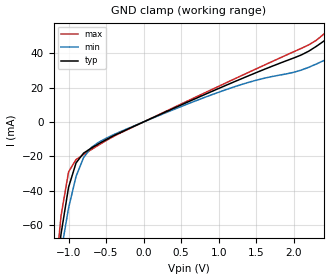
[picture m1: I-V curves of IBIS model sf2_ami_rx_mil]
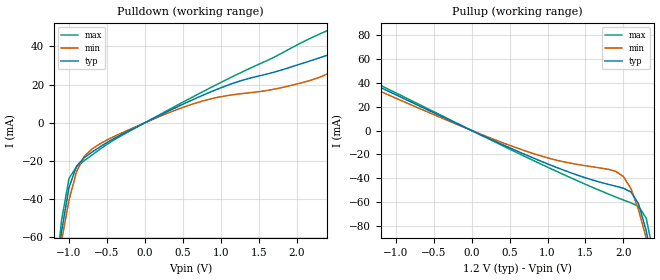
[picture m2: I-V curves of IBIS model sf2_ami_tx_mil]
|   Microsemi Corporation
|   SmarFusion2/IGLOO2 Military IBIS-AMI Models
[IBIS ver]   5.0
[File name]   sf2_igl2_ami_mil.ibs
[File Rev]   1.3
[Date]   February 1, 2019
[Disclaimer] These IBIS Models are Provided "As is" with NO WARRANTY
   whatsoever and signal integrity software specifically disclaims any
   implied warranties of merchantability, fitness for a particular
   purpose or against infringement.
[Source]   Original model developed in collaboration with Sigrity. Optimized by SiSoft.
[Notes]   Known limitations: Main tap is limited to maximum amplitude setting only
   and cannot be adjusted.
-Revision History:
1.4: February 1, 2019
   * Added model limitation note on abicdr_tx.ami and sf2_igl2_ami_mil.ibs files.
1.3: July 22, 2015
   * Added Algorithmic Model to support 64-bit Window environment
1.2: April 2, 2015
   * Added new RLC packages in Package section.
1.1: June 12, 2014
   * Updated Package section.
   * Consolidated the IGLOO2 and SmartFusion2 IBIS AMI Model
   * Updated the RX .ami model to clarify comments.
1.05: 6 November 2013
   Based on the model 1.0 model supplied by Microsemi dated 18 March 2013.
   This model has been optimized for use with SiSoft's QCD Simulator. Points of note:
   * Updated [Ramp] data to correct single-ended / differential issues
   * Updated C_comp values using data provided by Microsemi
   * Updated TX .ami file to disable auto EQ mode (does not work with QCD)
   * Included TX jitter data derived from PCIe Gen2 compliance testing
   * Signed models as QCD Certified
1.0: 18 March 2013 20:52:13
   * Original model supplied by Microsemi
[Copyright]  (c) 2013, Microsemi Corporation, All Rights Reserved.
[Component]  SF2_IGL2_ibis_ami_mil
[Manufacturer] Microsemi Corporation
[Package]
|   typ   min   max
| M2S/M2GL010
|R_pkg   0.66635   0.053835   1.0211   |010-FG484
|L_pkg   5.248e-9   6.178e-10   7.432e-9   |010-FG484
|C_pkg   1.306e-12   8.624e-13   3.748e-12   |010-FG484
| M2S/M2GL025
|R_pkg   0.62161   0.045855   0.88864   |025-FG484
|L_pkg   4.896e-9   4.955e-10   6.635e-9   |025-FG484
|C_pkg   1.283e-12   7.336e-13   4.781e-12   |025-FG484
| M2S/M2GL050
R_pkg   0.64708   0.10714   1.1617   |050-FG484
L_pkg   4.885e-9   8.618e-10   8.001e-9   |050-FG484
C_pkg   1.224e-12   7.009e-13   2.089e-12   |050-FG484
| M2S/M2GL060
|R_pkg   0.56892   0.053004   0.79188   |060-FG484
|L_pkg   4.842e-9   5.148e-10   6.754e-9   |060-FG484
|C_pkg   1.575e-12   9.705e-13   7.459e-12   |060-FG484
| M2S/M2GL090
|R_pkg   0.64363   0.064239   0.93501   |090-FG484
|L_pkg   4.937e-9   6.079e-10   6.828e-9   |090-FG484
|C_pkg   1.588e-12   6.307e-13   1.263e-11   |090-FG484
| M2S/M2GL150
|R_pkg   0.86225   0.11212   1.7907   |150-FC1152
|L_pkg   3.847e-9   9.122e-10   7.188e-9   |150-FC1152
|C_pkg   2.093e-12   9.047e-13   3.356e-12   |150-FC1152
| The PIN numbers given below are examples. They do not correspond to
| device pin numbers.
[Pin]   signal_name   model_name   R_pin  L_pin  C_pin
1p   sf2_tx_p   sf2_ami_tx_mil   NA   NA   NA
1n   sf2_tx_n   sf2_ami_tx_mil   NA   NA   NA
2p   sf2_rx_p   sf2_ami_rx_mil   NA   NA   NA
2n   sf2_rx_n   sf2_ami_rx_mil   NA   NA   NA
[Diff_Pin] inv_pin vdiff tdelay_typ tdelay_min tdelay_max
1p   1n   0.1V  NA   NA   NA
2p   2n   0.1V  NA   NA   NA
| Models and submodels in the file (2): sf2_ami_rx_mil (Input), sf2_ami_tx_mil (Output)
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|   Model sf2_ami_rx_mil
[Model] sf2_ami_rx_mil
|SiSoft ModelSignature1 b472d6ce902416eafb5b33f9e1345f04cfe18a74956e470ca32caceb1da95d23 Certified
Model_type Input
C_comp 0.914p 0.471p 1.37p
Vinh = 0.55
Vinl = 0.45
| Differential package model for post-route analysis
|SiSoft Diff_Package SF2_FG896_472673AP0A_0308_PCIE2_TxRx.s4p.smod s_SF2_FG896_472673AP0A_0308_PCIE2_TxRx
[Algorithmic Model]
Executable Windows_VisualStudio7.1.3088_32 abicdr_rx.dll   abicdr_rx.ami
Executable Windows_VisualStudio7.1.3088_64 abicdr_x64_rx.dll  abicdr_rx.ami
Executable Linux_gcc3.2.3_64   abicdr_rh64_rx.dll abicdr_rx.ami
[End Algorithmic Model]
[Temperature Range]   25C   125C   -55C
[Voltage Range]   1.2V   1.14V   1.26V
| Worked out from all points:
|   GND clamp passes 1 mA (typ) near -0.05 V on its own axis
[GND Clamp]
|Voltage   I(typ)   I(min)   I(max)
-2.5V     -710.8mA   -585.6mA   -919mA
-1.2V     -101.9mA   -106.1mA   -100.5mA
-1.1V     -65.27mA   -75.8mA    -54.63mA
-1V       -38.09mA   -50.18mA   -29.12mA
-900mV    -23.87mA   -31.72mA   -21.92mA
-800mV    -18.2mA    -20.83mA   -18.98mA
-700mV    -15.32mA   -15.03mA   -16.22mA
-600mV    -12.78mA   -11.88mA   -13.51mA
100mV     1.987mA    1.824mA    2.09mA
1V        19.46mA    17.27mA    20.72mA
2.2V      41.17mA    31.79mA    44.83mA
2.5V      50.17mA    37.82mA    55.2mA
|   Model sf2_ami_tx_mil
[Model] sf2_ami_tx_mil
|SiSoft ModelSignature1 d09a95125635bb18c3a6f7f6574f2fc09c04016d4fd52b13c486b8fdf58bb3a5 Certified
Model_type Output
C_comp 0.914p 0.471p 1.37p
Cref = 0
Vref = 0.5
Rref = 50
Vmeas = 0.6
| Differential package model for post-route analysis
|SiSoft Diff_Package SF2_FG896_472673AP0A_0308_PCIE2_TxRx.s4p.smod s_SF2_FG896_472673AP0A_0308_PCIE2_TxRx
[Algorithmic Model]
Executable Windows_VisualStudio7.1.3088_32 abicdr_tx.dll   abicdr_tx.ami
Executable Windows_VisualStudio7.1.3088_64 abicdr_x64_tx.dll  abicdr_tx.ami
Executable Linux_gcc3.2.3_64   abicdr_rh64_tx.dll abicdr_tx.ami
[End Algorithmic Model]
[Temperature Range]   25C   125C   -55C
[Voltage Range]   1.2V   1.14V   1.26V
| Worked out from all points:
|   slope of the pulldown table from 0 to 0.18 V, typ, clamps not added: 50.4 ohm
|   slope of the pullup table from 0 to 0.18 V, typ, clamps not added: 34.2 ohm
[Pulldown]
|Voltage   I(typ)   I(min)   I(max)
-2.5V     -663.6mA   -535.6mA   -873.7mA
-1.2V     -90.34mA   -89.14mA   -93.67mA
-1.1V     -57.52mA   -62.43mA   -51.53mA
-1V       -33.95mA   -40.47mA   -29.14mA
-900mV    -22.69mA   -25.54mA   -23.01mA
-800mV    -18.27mA   -17.71mA   -19.89mA
-600mV    -12.82mA   -11.22mA   -14.05mA
100mV     1.995mA    1.723mA    2.182mA
700mV     13.31mA    10.7mA     14.97mA
1.2V      21.19mA    14.92mA    25.04mA
1.9V      28.88mA    19.31mA    38.53mA
2.5V      36.63mA    27.48mA    49.9mA
[Pullup]
|Voltage   I(typ)   I(min)   I(max)
-3.7V     173.4mA    162.2mA    188.3mA
-2.7V     88.71mA    88.6mA     87.4mA
-1.9V     57.14mA    53.33mA    59.63mA
-100mV    2.954mA    2.608mA    3.146mA
1V        -27.86mA   -22.82mA   -30.6mA
1.9V      -46.55mA   -34.12mA   -55.56mA
2V        -48.22mA   -38.42mA   -58.05mA
2.1V      -51.37mA   -48.68mA   -60.46mA
2.2V      -61.31mA   -66.37mA   -63.34mA
2.3V      -83.51mA   -89.64mA   -73.16mA
2.4V      -114.9mA   -116.4mA   -103.7mA
3.6V      -622.5mA   -520.6mA   -796mA
[Ramp]
| variable   typ   min   max
dV/dt_r 0.3912/8.652e-11   0.3423/9.022e-11   0.4256/9.625e-11
dV/dt_f 0.3912/7.387e-11   0.3423/7.781e-11   0.4256/7.198e-11
R_load = 50
|End [Model] sf2_ami_tx_mil
|End [Component]
